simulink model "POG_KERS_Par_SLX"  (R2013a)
settings: Solver=ode45  StartTime=0.0  StopTime=10.0  MaxStep=0.001  RelTol=1e-3
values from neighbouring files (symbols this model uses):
  b_1 = 0    [POG_KERS_Par_SLX_m.m]    (also in POG_KERS_SLX_m.m = 1)
  b_2 = 0    [POG_KERS_Par_SLX_m.m]    (also in POG_KERS_SLX_m.m = 1)
  b_3 = 0    [POG_KERS_Par_SLX_m.m]    (also in POG_KERS_SLX_m.m = 1)
  b_b = 0    [POG_KERS_Par_SLX_m.m]    (also in POG_KERS_SLX_m.m = 1)
  J_1 = 0.026*kg*meters^2    [POG_KERS_Par_SLX_m.m]    (also in POG_KERS_SLX_m.m = 13)
  J_2 = 0.675*kg*r_2^2    [POG_KERS_Par_SLX_m.m]    (also in POG_KERS_SLX_m.m = 1)
  J_3 = 100*J_2    [POG_KERS_Par_SLX_m.m]    (also in POG_KERS_SLX_m.m = 1)
  J_b = 1.0*kg*r_b^2    [POG_KERS_Par_SLX_m.m]    (also in POG_KERS_SLX_m.m = 1)
  K_1_2 = Inf    (= inf)    [POG_KERS_EQN_Reduced.m]    (also in POG_KERS_Par_SLX_m.m = 150*Newton/(0.2*mm); POG_KERS_SLX_m.m = 1)
  K_2_b = Inf    (= inf)    [POG_KERS_EQN_Reduced.m]    (also in POG_KERS_Par_SLX_m.m = 80*Newton/(0.2*mm); POG_KERS_SLX_m.m = 1)
  K_b_3 = Inf    (= inf)    [POG_KERS_EQN_Reduced.m]    (also in POG_KERS_Par_SLX_m.m = 80*Newton/(0.2*mm); POG_KERS_SLX_m.m = 1)
  r_1 = 17.2*mm    [POG_KERS_Par_SLX_m.m]    (also in POG_KERS_SLX_m.m = 1)
  r_2 = 51.5*mm    [POG_KERS_Par_SLX_m.m]    (also in POG_KERS_SLX_m.m = 1)
  r_a = 34.3*mm    [POG_KERS_Par_SLX_m.m]
  r_b = 27.5*mm    [POG_KERS_Par_SLX_m.m]    (also in POG_KERS_SLX_m.m = 1)
  T_1_0 = 0*Nm    [POG_KERS_Par_SLX_m.m]    (also in POG_KERS_SLX_m.m = 0)
  Ts = Tfin/Nr_Ts_Points    (= 0.0015)    [POG_KERS_Par_SLX_m.m]    (also in POG_KERS_SLX_m.m = 0.005)
  w_1_0 = 2000*rpm    [POG_KERS_Par_SLX_m.m]
  w_2_0 = w_1_0*r_1/r_2    [POG_KERS_Par_SLX_m.m]
  w_3_0 = w_b_0*r_b/r_3_t_h    [POG_KERS_Par_SLX_m.m]
  w_b_0 = w_2_0*r_2_t_h/r_b    [POG_KERS_Par_SLX_m.m]
  x_1_3_0 = 0    [POG_KERS_Par_SLX_m.m]    (also in POG_KERS_SLX_m.m)
  x_2_0_0 = 0    [POG_KERS_Par_SLX_m.m]    (also in POG_KERS_SLX_m.m)
  x_6_0 = 0    [POG_KERS_Par_SLX_m.m]    (also in POG_KERS_SLX_m.m)

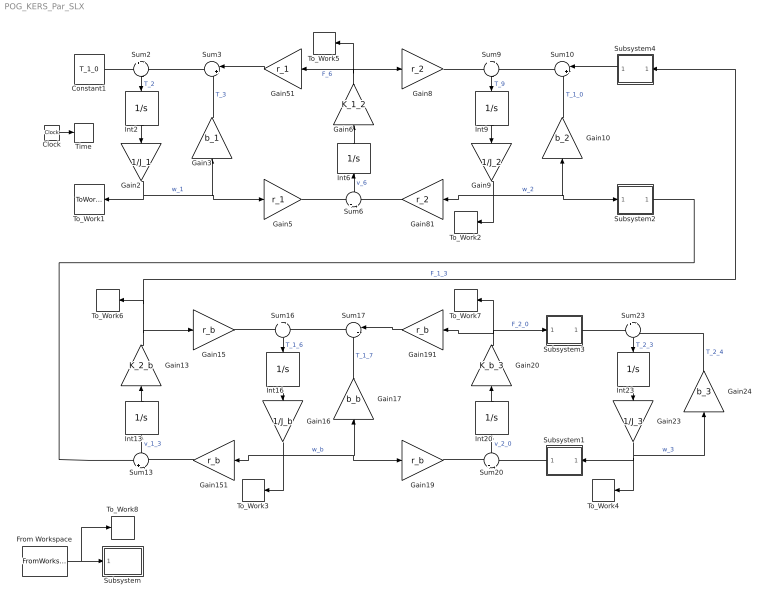
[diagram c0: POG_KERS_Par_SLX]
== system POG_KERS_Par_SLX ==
  Clock : Clock
  Constant1 : Constant  Value=T_1_0
  From Workspace : FromWorkspace  VariableName=[tt th]  SampleTime=0
  Gain10 : Gain  Gain=b_2  Multiplication=Matrix(K*u)
  Gain13 : Gain  Gain=K_2_b  Multiplication=Matrix(K*u)
  Gain{15,19,151,191} (4 alike) : Gain  Gain=r_b  Multiplication=Matrix(K*u)
  Gain16 : Gain  Gain=1/J_b  Multiplication=Matrix(K*u)
  Gain17 : Gain  Gain=b_b  Multiplication=Matrix(K*u)
  Gain2 : Gain  Gain=1/J_1  Multiplication=Matrix(K*u)
  Gain20 : Gain  Gain=K_b_3  Multiplication=Matrix(K*u)
  Gain23 : Gain  Gain=1/J_3  Multiplication=Matrix(K*u)
  Gain24 : Gain  Gain=b_3  Multiplication=Matrix(K*u)
  Gain3 : Gain  Gain=b_1  Multiplication=Matrix(K*u)
  Gain5 : Gain  Gain=r_1  Multiplication=Matrix(K*u)
  Gain51 : Gain  Gain=r_1  Multiplication=Matrix(K*u)
  Gain6 : Gain  Gain=K_1_2  Multiplication=Matrix(K*u)
  Gain8 : Gain  Gain=r_2  Multiplication=Matrix(K*u)
  Gain81 : Gain  Gain=r_2  Multiplication=Matrix(K*u)
  Gain9 : Gain  Gain=1/J_2  Multiplication=Matrix(K*u)
  Int13 : Integrator  InitialCondition=x_1_3_0
  Int16 : Integrator  InitialCondition=w_b_0*J_b
  Int2 : Integrator  InitialCondition=w_1_0*J_1
  Int20 : Integrator  InitialCondition=x_2_0_0
  Int23 : Integrator  InitialCondition=w_3_0*J_3
  Int6 : Integrator  InitialCondition=x_6_0
  Int9 : Integrator  InitialCondition=w_2_0*J_2
  Subsystem : Subsystem
  Subsystem1 : Subsystem
  Subsystem2 : Subsystem
  Subsystem3 : Subsystem
  Subsystem4 : Subsystem
  Sum10 : Sum  Inputs=|++
  Sum{2,6,9,13,16,20,23} (7 alike) : Sum  Inputs=+|-
  Sum17 : Sum  Inputs=|++
  Sum3 : Sum  Inputs=|++
  Time : ToWorkspace  VariableName=t  SampleTime=Ts
  To_Work1 : ToWorkspace  VariableName=w_1  SampleTime=Ts
  To_Work2 : ToWorkspace  VariableName=w_2  SampleTime=Ts
  To_Work3 : ToWorkspace  VariableName=w_b  SampleTime=Ts
  To_Work4 : ToWorkspace  VariableName=w_3  SampleTime=Ts
  To_Work5 : ToWorkspace  VariableName=f_1_2  SampleTime=Ts
  To_Work6 : ToWorkspace  VariableName=f_2_b  SampleTime=Ts
  To_Work7 : ToWorkspace  VariableName=f_b_3  SampleTime=Ts
  To_Work8 : ToWorkspace  VariableName=Th  SampleTime=Ts
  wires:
  Constant1/1 -> Sum2/1
  Sum3/1 -> Sum2/2
  Gain2/1 -> To_Work1/1, Gain3/1, Gain5/1  "w_1"
  Sum2/1 -> Int2/1  "T_2"
  Int2/1 -> Gain2/1
  Gain51/1 -> Sum3/1
  Gain3/1 -> Sum3/2  "T_3"
  Gain5/1 -> Sum6/1
  Gain6/1 -> To_Work5/1, Gain51/1, Gain8/1  "F_6"
  Gain81/1 -> Sum6/2
  Sum6/1 -> Int6/1  "v_6"
  Int6/1 -> Gain6/1
  Gain8/1 -> Sum9/1
  Gain9/1 -> To_Work2/1, Gain81/1, Subsystem2/1(In), Gain10/1  "w_2"
  Sum10/1 -> Sum9/2
  Sum9/1 -> Int9/1  "T_9"
  Int9/1 -> Gain9/1
  Subsystem4/1(Out) -> Sum10/1
  Gain10/1 -> Sum10/2  "T_1_0"
  Subsystem2/1(Out) -> Sum13/1
  Gain13/1 -> Subsystem4/1(In), To_Work6/1, Gain15/1  "F_1_3"
  Gain151/1 -> Sum13/2
  Sum13/1 -> Int13/1  "v_1_3"
  Int13/1 -> Gain13/1
  Gain15/1 -> Sum16/1
  Gain16/1 -> To_Work3/1, Gain151/1, Gain17/1, Gain19/1  "w_b"
  Sum17/1 -> Sum16/2
  Sum16/1 -> Int16/1  "T_1_6"
  Int16/1 -> Gain16/1
  Gain191/1 -> Sum17/1
  Gain17/1 -> Sum17/2  "T_1_7"
  Gain19/1 -> Sum20/1
  Gain20/1 -> To_Work7/1, Gain191/1, Subsystem3/1(In)  "F_2_0"
  Subsystem1/1(Out) -> Sum20/2
  Sum20/1 -> Int20/1  "v_2_0"
  Int20/1 -> Gain20/1
  Subsystem3/1(Out) -> Sum23/1
  Gain23/1 -> Subsystem1/1(In), To_Work4/1, Gain24/1  "w_3"
  Gain24/1 -> Sum23/2  "T_2_4"
  Sum23/1 -> Int23/1  "T_2_3"
  Int23/1 -> Gain23/1
  Clock/1 -> Time/1
  From Workspace/1 -> To_Work8/1, Subsystem/1(th)

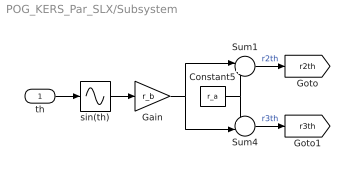
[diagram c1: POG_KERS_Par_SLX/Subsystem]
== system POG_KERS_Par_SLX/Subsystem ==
  th : Inport
  Constant5 : Constant  Value=r_a
  Gain : Gain  Gain=r_b
  Sum1 : Sum  Inputs=|++
  Sum4 : Sum  Inputs=+-|
  sin(th) : Sin  TimeSource=Use external signal  SampleTime=0
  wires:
  th/1 -> sin(th)/1
  sin(th)/1 -> Gain/1
  Sum4/1 -> [r3th]  "r3th"
  Gain/1 -> Sum4/2, Sum1/1
  Constant5/1 -> Sum4/1, Sum1/2
  Sum1/1 -> [r2th]  "r2th"

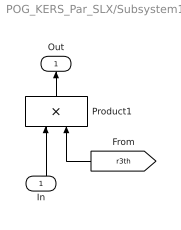
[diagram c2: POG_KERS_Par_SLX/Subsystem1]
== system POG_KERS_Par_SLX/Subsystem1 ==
  In : Inport
  Product1 : Product
  Out : Outport
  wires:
  Product1/1 -> Out/1
  In/1 -> Product1/1
  [r3th] -> Product1/2

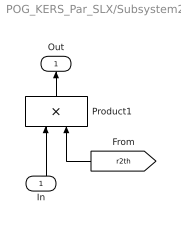
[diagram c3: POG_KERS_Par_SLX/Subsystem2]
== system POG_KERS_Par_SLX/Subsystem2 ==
  In : Inport
  Product1 : Product
  Out : Outport
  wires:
  Product1/1 -> Out/1
  In/1 -> Product1/1
  [r2th] -> Product1/2

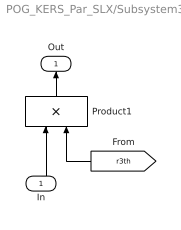
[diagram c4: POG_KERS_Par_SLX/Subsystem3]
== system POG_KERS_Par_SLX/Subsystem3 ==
  In : Inport
  Product1 : Product
  Out : Outport
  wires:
  [r3th] -> Product1/2
  In/1 -> Product1/1
  Product1/1 -> Out/1

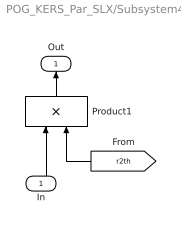
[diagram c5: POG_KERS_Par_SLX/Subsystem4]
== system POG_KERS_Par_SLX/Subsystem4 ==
  In : Inport
  Product1 : Product
  Out : Outport
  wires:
  [r2th] -> Product1/2
  In/1 -> Product1/1
  Product1/1 -> Out/1
